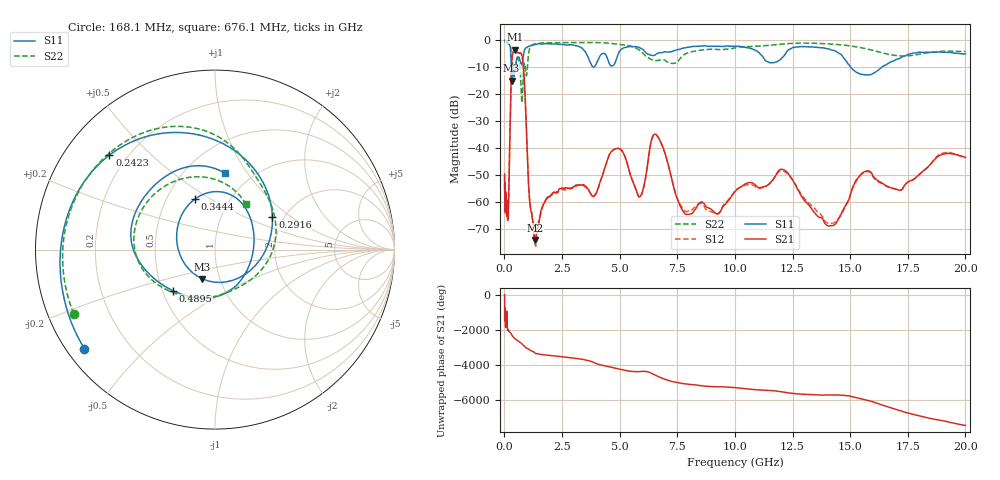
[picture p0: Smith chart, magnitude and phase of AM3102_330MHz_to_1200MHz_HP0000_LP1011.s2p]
! Date/Time: Tue, Sep 11, 2018 5:09 PM
! Network Analyzer: Agilent Technologies E8362B Rev: A.07.50.63
! Sweep from 0.010 to 20.000 GHz, 1601 Points, Sweep Type: LOG
! Power Supply: 4.950 V, 0.001 A
# Hz S DB R 50
!freq MagS11 AngS11 MagS21 AngS21 MagS12 AngS12 MagS22 AngS22
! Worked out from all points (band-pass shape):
!   1601 points, 10 MHz to 20 GHz, reference 50 ohm
!   highest |S21| = -3.48 dB at 447.2 MHz (marker M1); lowest = -74.3 dB at 1.334 GHz (marker M2)
!   |S21| within 3 dB of the highest: 331.2 MHz to 782.8 MHz (451.6 MHz wide, 81.1 % of centre)
!   lowest |S11| = -15.0 dB at 314.7 MHz (marker M3), VSWR 1.43, Z = 41.3 - j13.9 ohm
!   |S11| at or under -10 dB: 295.3 MHz to 349.3 MHz (53.99 MHz wide, 16.8 % of centre); 365.3 MHz to 485.1 MHz (119.9 MHz wide, 28.2 % of centre); 15.03 GHz to 16.37 GHz (1.347 GHz wide, 8.58 % of centre)
!   |S22| runs from -23.2 to -0.3 dB; largest |S21 - S12| = 0.012
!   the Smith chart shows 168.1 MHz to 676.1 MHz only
!   S11 on the Smith chart (normalised r, x): 168.1 MHz: 0.05, -0.34; 242.3 MHz: 0.13, +0.38; 291.6 MHz: 1.75, +0.73; 344.4 MHz: 0.69, +0.43; 489.5 MHz: 0.57, -0.29; 676.1 MHz: 0.76, +0.79
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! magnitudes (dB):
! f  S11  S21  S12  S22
! 10 MHz  0.0  -49.7  -50.4  -0.3
! 35.55 MHz  0.0  -61.5  -60.6  -0.5
! 126.4 MHz  -0.4  -62.1  -63.5  -1.1
! 168.1 MHz  -0.8  -65.8  -62.8  -1.3
! 242.3 MHz  -2.1  -34.2  -34.3  -1.8
! 291.6 MHz  -8.7  -13.8  -13.9  -3.6
! 314.7 MHz  -15.0  -8.3  -8.3  -5.8
! 344.4 MHz  -10.4  -5.7  -5.8  -8.0
! 447.2 MHz  -12.1  -3.5  -3.5  -11.1
! 489.5 MHz  -9.7  -3.6  -3.7  -9.1
! 676.1 MHz  -7.3  -4.7  -4.7  -10.3
! 841.2 MHz  -4.7  -11.7  -11.8  -10.4
! 1.334 GHz  -1.5  -74.3  -76.1  -1.3
! 1.59 GHz  -1.4  -63.3  -63.9  -1.0
! 3.902 GHz  -9.8  -57.9  -57.7  -0.8
! 4.855 GHz  -7.1  -40.3  -40.3  -1.3
! 5.652 GHz  -2.3  -54.2  -54.3  -2.6
! 6.612 GHz  -4.9  -35.3  -35.4  -7.5
! 7.882 GHz  -2.7  -64.8  -63.7  -4.9
! 12.09 GHz  -6.1  -48.1  -48.5  -1.3
! 14.07 GHz  -3.2  -69.1  -68.1  -1.3
! 20 GHz  -5.1  -43.5  -43.9  -4.1
